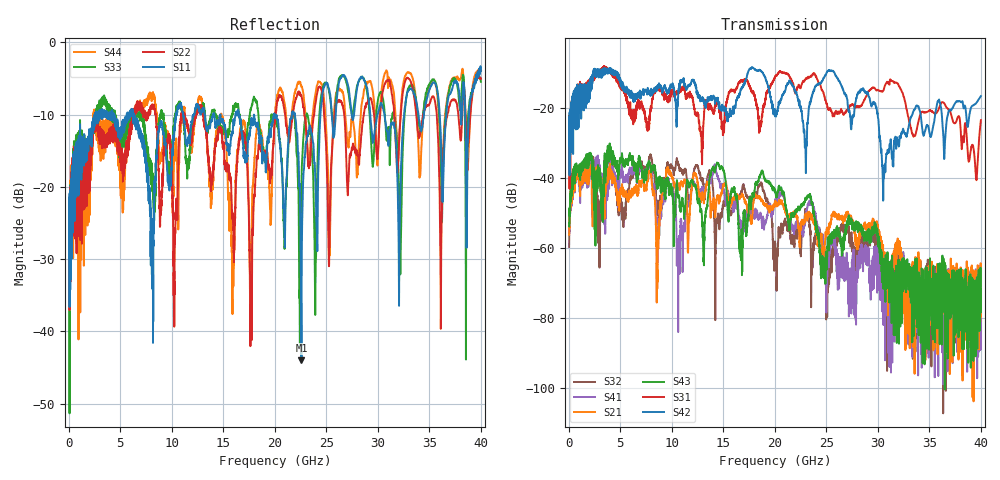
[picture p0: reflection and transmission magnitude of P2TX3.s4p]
!Agilent Technologies,N5245A,MY49151084,A.09.20.08
!Agilent N5245A: A.09.20.08
!Date: Thursday, March 01, 2012 14:15:45
!Correction: S11(Full 4 Port(1,2,3,4))
!S12(Full 4 Port(1,2,3,4))
!S13(Full 4 Port(1,2,3,4))
!S14(Full 4 Port(1,2,3,4))
!S21(Full 4 Port(1,2,3,4))
!S22(Full 4 Port(1,2,3,4))
!S23(Full 4 Port(1,2,3,4))
!S24(Full 4 Port(1,2,3,4))
!S31(Full 4 Port(1,2,3,4))
!S32(Full 4 Port(1,2,3,4))
!S33(Full 4 Port(1,2,3,4))
!S34(Full 4 Port(1,2,3,4))
!S41(Full 4 Port(1,2,3,4))
!S42(Full 4 Port(1,2,3,4))
!S43(Full 4 Port(1,2,3,4))
!S44(Full 4 Port(1,2,3,4))
!S4P File: Measurements: <S11,S12,S13,S14>,
!<S21,S22,S23,S24>,
!<S31,S32,S33,S34>,
!<S41,S42,S43,S44>:
# Hz S  dB  R 50
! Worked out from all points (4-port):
!   3996 points, 50 MHz to 40 GHz, reference 50 ohm
!   strongest paths, dB at 50 MHz, 10.04 GHz, 20.03 GHz, 30.02 GHz, 40 GHz:
!     S42: -26.9, -13.5, -21.7, -22.9, -16.6
!     S31: -25.5, -15.5, -11.1, -14.9, -23.5
!     S43: -53.6, -43.4, -43.4, -55.9, -71.6
!     S21: -56.1, -39.8, -46.7, -56.2, -70.8
!     S41: -55.6, -43.1, -46.1, -65.9, -72.8
!     S32: -59.6, -37.1, -58.0, -58.5, -78.2
!   lowest |S11| = -44.0 dB at 22.59 GHz (marker M1), VSWR 1.01, Z = 49.9 + j0.615 ohm
!   |S11| at or under -10 dB: start of sweep to 2.53 GHz; 6.36 GHz to 10.45 GHz (4.087 GHz wide, 48.6 % of centre); 21.96 GHz to 24.43 GHz (2.464 GHz wide, 10.6 % of centre)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
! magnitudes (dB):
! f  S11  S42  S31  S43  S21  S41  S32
! 50 MHz  -23.5  -26.9  -25.5  -53.6  -56.1  -55.6  -59.6
! 7.93 GHz  -22.1  -16.1  -21.1  -36.2  -38.2  -37.1  -33.3
! 10.64 GHz  -9.1  -15.9  -15.3  -45.6  -42.4  -68.1  -36.0
! 17.71 GHz  -10.9  -8.7  -14.6  -48.3  -53.1  -51.1  -47.1
! 22.59 GHz  -44.0  -20.7  -13.4  -47.5  -52.7  -54.7  -58.3
! 30.59 GHz  -9.6  -38.5  -14.5  -63.0  -62.6  -71.0  -64.7
! 40 GHz  -4.0  -16.6  -23.5  -71.6  -70.8  -72.8  -78.2
